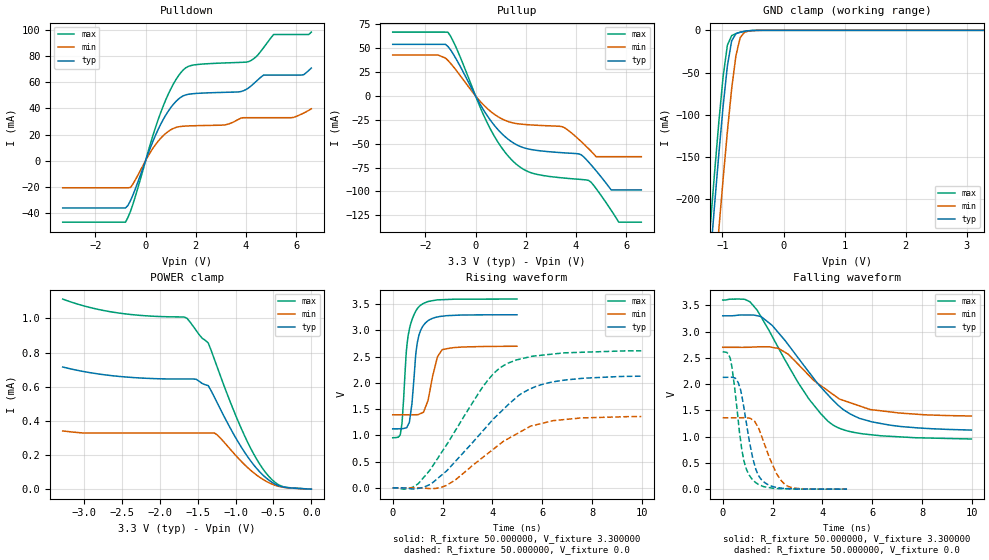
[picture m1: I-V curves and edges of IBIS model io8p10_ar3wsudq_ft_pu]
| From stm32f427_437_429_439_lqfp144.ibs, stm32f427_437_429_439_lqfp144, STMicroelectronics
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|   Model io8p10_ar3wsudq_ft_pu
[Model]  io8p10_ar3wsudq_ft_pu
Model_type I/O
Polarity   Non-Inverting
Enable   Active-Low
Vinl =   0.990000V
Vinh =   2.310000V
Vmeas =  1.650000V
Cref =   40.000000pF
Rref =   100.000000M
Vref =   0.0V
C_comp   3.843100pF   3.761700pF   3.937000pF
[Temperature Range]   25.000000   0.125000k   -40.000000
[Pullup Reference]   3.300000V   2.700000V   3.600000V
[Pulldown Reference]   0.0V   0.0V   0.0V
[POWER Clamp Reference]   3.300000V   2.700000V   3.600000V
[GND Clamp Reference]   0.0V   0.0V   0.0V
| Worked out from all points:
|   slope of the pulldown table from 0 to 0.495 V, typ, clamps not added: 20.9 ohm
|   slope of the pullup table from 0 to 0.495 V, typ, clamps not added: 22.6 ohm
|   GND clamp passes 1 mA (typ) near -0.62 V on its own axis
|   rising waveform, R_fixture 50.000000, V_fixture 3.300000: 20-80 % time 272ps typ, 357ps min, 282ps max; typ from 1.12 V to 3.3 V
|   rising waveform, R_fixture 50.000000, V_fixture 0.0: 20-80 % time 2.55ns typ, 2.37ns min, 2.13ns max; typ from 0.001 V to 2.13 V
|   falling waveform, R_fixture 50.000000, V_fixture 3.300000: 20-80 % time 2.28ns typ, 2.16ns min, 2.06ns max; typ from 3.3 V to 1.12 V
|   falling waveform, R_fixture 50.000000, V_fixture 0.0: 20-80 % time 505ps typ, 695ps min, 425ps max; typ from 2.13 V to 0.001 V
[Pulldown]
|Voltage   I(typ)   I(min)   I(max)
-3.3V     -36.18mA   -20.77mA   -47.07mA
-800mV    -36.18mA   -20.77mA   -47.07mA
-600mV    -30.5mA    -20.52mA   -38.69mA
700mV     31.4mA     19.11mA    41.71mA
1.2V      45.15mA    25.37mA    61.75mA
1.6V      50.35mA    26.5mA     71.06mA
3.1V      52.28mA    27.26mA    74.76mA
4.1V      55.65mA    32.89mA    75.79mA
4.7V      65.5mA     32.89mA    86.49mA
5.1V      65.5mA     32.89mA    96.55mA
6.3V      65.83mA    36.49mA    96.55mA
6.6V      70.88mA    39.7mA     98.4mA
[Pullup]
|Voltage   I(typ)   I(min)   I(max)
-3.3V     54.05mA    42.9mA     66.88mA
-1.1V     51.84mA    37.22mA    66.67mA
500mV     -22.06mA   -14mA      -30.03mA
1.5V      -49.1mA    -28.3mA    -68.56mA
2.2V      -56.04mA   -30.32mA   -80.35mA
3.5V      -59.52mA   -32.72mA   -85.91mA
4.2V      -61.52mA   -47.62mA   -87.45mA
4.5V      -69.2mA    -55.26mA   -88.43mA
4.8V      -78.37mA   -63.6mA    -97mA
5.4V      -98.4mA    -63.6mA    -119.7mA
5.7V      -98.4mA    -63.6mA    -132.2mA
6.6V      -98.4mA    -63.6mA    -132.2mA
[GND_clamp]
|Voltage   I(typ)   I(min)   I(max)
-3.3V     -2.327A    -2.405A    -2.301A
-1.2V     -270.2mA   -361.4mA   -232.1mA
-1.13V    -207.3mA   -298.1mA   -169mA
-1.06V    -146.7mA   -236.2mA   -108.8mA
-990mV    -90.18mA   -176.4mA   -54.96mA
-920mV    -42.21mA   -120mA     -17.68mA
-850mV    -12.57mA   -69.47mA   -6.265mA
-780mV    -3.971mA   -30.01mA   -3.886mA
-710mV    -2.1mA     -8.615mA   -2.382mA
-640mV    -1.148mA   -2.283mA   -1.22mA
-570mV    -524uA     -821.5uA   -476.8uA
3.28V     0A         0A         0A
[POWER_clamp]
|Voltage   I(typ)   I(min)   I(max)
-3.28V    715.1uA    340.8uA    1.113mA
-2.6V     662.9uA    328.8uA    1.035mA
-1.64V    645uA      328.8uA    1mA
-1.52V    643.3uA    328.8uA    929.5uA
-1.36V    606.3uA    328.8uA    855.6uA
-1.24V    503.7uA    316.8uA    712.3uA
-960mV    272.5uA    179.4uA    391.9uA
-800mV    165.1uA    110.4uA    239.2uA
-640mV    83.2uA     57.57uA    119.3uA
-520mV    40.52uA    29.83uA    56.09uA
-400mV    15.54uA    13.29uA    18.7uA
0V        0A         0A         0A
[Ramp]
| variable   typ   min   max
dV/dt_r  1.26673/2.54659n   0.81111/2.37409n   1.56382/2.13375n
dV/dt_f  1.28190/2.27080n   0.77550/2.14553n   1.57403/2.05442n
R_load = 50.000000
[Rising Waveform]
R_fixture= 50.000000
V_fixture= 3.300000
V_fixture_min= 2.700000
V_fixture_max= 3.600000
|time   V(typ)   V(min)   V(max)
0s        1.125V     1.393V     955.6mV
300.3ps   1.127V     1.393V     1.008V
370.4ps   1.128V     1.393V     1.221V
550.6ps   1.145V     1.393V     2.621V
670.7ps   1.257V     1.393V     3.031V
1.031ns   2.865V     1.399V     3.443V
1.411ns   3.185V     1.661V     3.551V
1.792ns   3.258V     2.494V     3.584V
1.982ns   3.272V     2.634V     3.587V
4.985ns   3.3V       2.7V       3.599V
[Rising Waveform]
R_fixture= 50.000000
V_fixture= 0.0
V_fixture_min= 0.0
V_fixture_max= 0.0
|time   V(typ)   V(min)   V(max)
0s        1.432mV    1.24mV     1.813mV
480.5ps   -1.451mV   1.18mV     -23.36mV
1.021ns   -10.1mV    -415.6uV   77.63mV
1.522ns   68.96mV    -14.26mV   358mV
2.142ns   315.5mV    44.32mV    808.2mV
3.644ns   1.102V     592mV      1.945V
4.484ns   1.519V     899.5mV    2.342V
5.185ns   1.804V     1.086V     2.464V
6.266ns   2.005V     1.262V     2.543V
9.97ns    2.129V     1.359V     2.612V
[Falling Waveform]
R_fixture= 50.000000
V_fixture= 3.300000
V_fixture_min= 2.700000
V_fixture_max= 3.600000
|time   V(typ)   V(min)   V(max)
0s        3.3V       2.7V       3.599V
1.101ns   3.315V     2.702V     3.563V
1.542ns   3.285V     2.71V      3.277V
2.242ns   2.973V     2.678V     2.683V
2.623ns   2.754V     2.57V      2.358V
3.463ns   2.225V     2.162V     1.713V
4.484ns   1.665V     1.783V     1.205V
5.125ns   1.429V     1.644V     1.095V
5.986ns   1.281V     1.512V     1.035V
9.97ns    1.125V     1.393V     955.6mV
[Falling Waveform]
R_fixture= 50.000000
V_fixture= 0.0
V_fixture_min= 0.0
V_fixture_max= 0.0
|time   V(typ)   V(min)   V(max)
0s        2.129V     1.359V     2.612V
300.3ps   2.13V      1.359V     2.491V
470.5ps   2.118V     1.359V     1.963V
620.6ps   2.031V     1.359V     1.319V
850.9ps   1.548V     1.361V     540.8mV
1.201ns   600.2mV    1.319V     181.2mV
1.592ns   164.4mV    966.1mV    59.02mV
2.162ns   34.09mV    294.9mV    12.95mV
2.472ns   14.56mV    102.6mV    8.938mV
4.985ns   1.432mV    1.24mV     1.813mV
